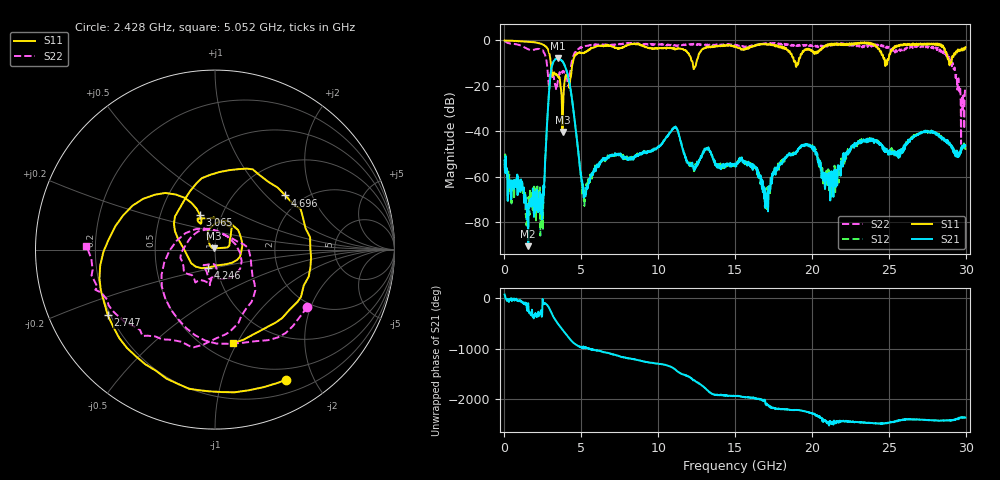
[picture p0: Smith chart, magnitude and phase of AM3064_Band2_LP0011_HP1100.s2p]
# Hz S DB R 50.0
!freq dBS11 angS11 dBS21 angS21 dBS12 angS12 dBS22 angS22
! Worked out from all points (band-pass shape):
!   1600 points, 10 MHz to 29.98 GHz, reference 50 ohm
!   highest |S21| = -7.89 dB at 3.459 GHz (marker M1); lowest = -90.6 dB at 1.547 GHz (marker M2)
!   |S21| within 3 dB of the highest: 3.099 GHz to 3.904 GHz (805.5 MHz wide, 23 % of centre)
!   lowest |S11| = -40.3 dB at 3.777 GHz (marker M3), VSWR 1.02, Z = 49.4 + j0.742 ohm
!   |S11| at or under -10 dB: 3.017 GHz to 4.443 GHz (1.427 GHz wide, 38.2 % of centre); 12.25 GHz to 12.48 GHz (229.5 MHz wide, 1.86 % of centre); 18.93 GHz to 19.11 GHz (182.4 MHz wide, 0.959 % of centre)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
!   |S22| runs from -45.6 to -0.2 dB; largest |S21 - S12| = 0.013
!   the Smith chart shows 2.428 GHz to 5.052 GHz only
!   S11 on the Smith chart (normalised r, x): 2.428 GHz: 0.35, -1.63; 2.747 GHz: 0.19, -0.27; 3.065 GHz: 0.79, +0.32; 4.246 GHz: 0.91, -0.18; 4.696 GHz: 1.64, +1.31; 5.052 GHz: 0.67, -0.97
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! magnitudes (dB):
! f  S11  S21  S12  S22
! 10 MHz  0.0  -52.9  -54.2  -0.2
! 1.547 GHz  -0.6  -90.6  -73.0  -3.9
! 2.428 GHz  -1.7  -68.8  -76.6  -4.4
! 2.747 GHz  -3.1  -39.9  -39.5  -9.6
! 3.065 GHz  -13.4  -11.9  -11.9  -15.7
! 3.459 GHz  -15.5  -7.9  -8.1  -18.3
! 3.777 GHz  -40.3  -9.3  -9.4  -14.3
! 4.246 GHz  -19.4  -19.2  -19.4  -14.8
! 4.696 GHz  -6.1  -42.7  -42.8  -4.6
! 5.015 GHz  -5.7  -62.2  -59.7  -3.2
! 5.052 GHz  -5.5  -61.8  -67.5  -2.8
! 10 GHz  -3.5  -46.7  -46.9  -1.8
! 11.09 GHz  -4.1  -38.2  -38.3  -2.0
! 12.25 GHz  -10.2  -55.1  -55.0  -1.9
! 15 GHz  -2.6  -55.0  -55.5  -1.9
! 17.03 GHz  -1.8  -68.8  -73.6  -1.3
! 19.99 GHz  -4.3  -47.0  -46.8  -2.1
! 21.28 GHz  -1.7  -60.1  -65.3  -1.6
! 23.03 GHz  -1.3  -44.8  -45.6  -2.7
! 25 GHz  -8.0  -48.6  -49.1  -2.9
! 28.56 GHz  -3.1  -43.6  -43.0  -4.7
! 29.98 GHz  -3.0  -46.4  -48.2  -21.7
